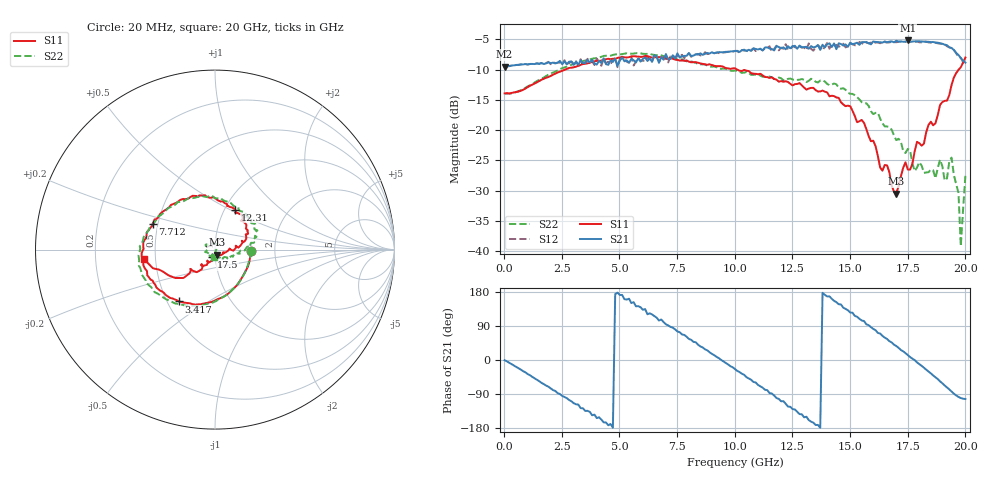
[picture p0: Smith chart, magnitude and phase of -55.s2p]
!Agilent Technologies,N5230A,US43500223,A.07.50.48
!Agilent N5230A: A.07.50.48
!Date: Monday, September 14, 2015 16:14:16
!Correction: S11(Full 2 Port(1,2))
!S21(Full 2 Port(1,2))
!S12(Full 2 Port(1,2))
!S22(Full 2 Port(1,2))
!S2P File: Measurements: S11, S21, S12, S22:
# Hz S  dB  R 50
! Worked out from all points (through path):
!   201 points, 20 MHz to 20 GHz, reference 50 ohm
!   highest |S21| = -5.18 dB at 17.5 GHz (marker M1); lowest = -9.5 dB at 20 MHz (marker M2)
!   group delay of S21, straight-line fit = 114 ps
!   lowest |S11| = -30.5 dB at 17 GHz (marker M3), VSWR 1.06, Z = 50.9 - j2.85 ohm
!   |S11| at or under -10 dB: start of sweep to 2.639 GHz; 10.1 GHz to 19.71 GHz (9.607 GHz wide, 64.4 % of centre)
!   |S22| runs from -39.2 to -7.3 dB; largest |S21 - S12| = 0.073
!   S11 on the Smith chart (normalised r, x): 20 MHz: 1.50, -0.02; 3.417 GHz: 0.57, -0.38; 7.712 GHz: 0.47, +0.16; 12.31 GHz: 1.12, +0.53; 17.5 GHz: 0.96, -0.08; 20 GHz: 0.43, -0.06
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2e7  -13.93 -1.9  -9.49 -0.6  -9.52 -0.5  -13.98 -1.6
1.9181e9  -11.22 -85.7  -8.79 -70.4  -8.71 -70.7  -10.83 -89.0
3.4166e9  -9.08 -124.8  -8.89 -127.4  -9.33 -130.0  -8.57 -126.3
5.1149e9  -7.88 -159.3  -7.97 171.7  -8.15 170.1  -7.43 -157.9
6.7133e9  -7.92 174.6  -8.87 104.1  -8.72 103.9  -7.54 177.4
7.7123e9  -8.48 157.5  -7.80 67.3  -7.55 66.7  -8.30 159.8
1.001e10  -9.77 112.4  -6.93 -24.2  -6.89 -24.8  -10.15 105.2
1.15085e10  -11.39 83.1  -6.50 -87.5  -6.13 -86.3  -11.15 72.8
1.23077e10  -12.04 63.4  -6.13 -123.0  -6.57 -121.0  -11.53 52.1
1.34066e10  -13.01 38.6  -6.33 -165.3  -6.88 -167.3  -11.63 31.1
1.4006e10  -13.77 25.6  -5.81 167.8  -5.57 168.8  -12.35 21.7
1.55045e10  -18.32 9.0  -5.44 104.2  -5.61 103.4  -15.39 0.7
1.67033e10  -26.99 -44.2  -5.37 49.7  -5.50 50.2  -19.48 -19.1
1.7003e10  -30.52 -70.0  -5.24 36.9  -5.48 36.3  -21.65 -34.7
1.75025e10  -26.53 -114.4  -5.18 13.1  -5.37 12.7  -23.10 -53.9
1.87013e10  -18.86 -126.8  -5.51 -45.6  -5.57 -46.2  -27.98 -144.0
1.89011e10  -15.84 -128.7  -5.64 -56.4  -5.72 -57.2  -24.88 -165.6
1.91009e10  -15.16 -142.1  -5.87 -67.2  -5.81 -68.1  -28.32 172.9
1.94006e10  -12.53 -138.0  -6.42 -83.1  -6.51 -83.7  -24.55 152.2
1.97003e10  -10.05 -157.1  -7.57 -97.4  -7.90 -99.5  -30.39 69.0
1.98002e10  -9.61 -160.2  -8.11 -100.4  -8.04 -100.8  -39.19 38.1
2e10  -8.00 -172.2  -8.85 -103.0  -9.13 -105.7  -27.55 -99.5
